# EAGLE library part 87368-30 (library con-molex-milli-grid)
RECEPTACAL
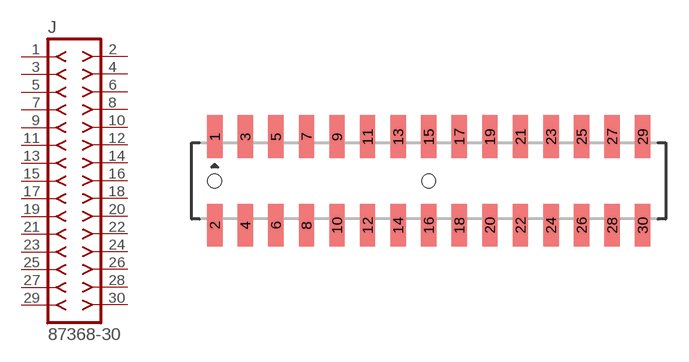
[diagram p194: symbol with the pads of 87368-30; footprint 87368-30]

Designator prefix J

## 87368-30  [87368-30]
1  1  pas
2  2  pas
3  3  pas
4  4  pas
5  5  pas
6  6  pas
7  7  pas
8  8  pas
9  9  pas
10  10  pas
11  11  pas
12  12  pas
13  13  pas
14  14  pas
15  15  pas
16  16  pas
17  17  pas
18  18  pas
19  19  pas
20  20  pas
21  21  pas
22  22  pas
23  23  pas
24  24  pas
25  25  pas
26  26  pas
27  27  pas
28  28  pas
29  29  pas
30  30  pas

## Footprint 87368-30 (pad centres in mm)
RECEPTACAL SMD Dual Row, Side Entry
smd 1 x 2.8: 1 -14,2.9; 2 -14,-2.9; 3 -12,2.9; 4 -12,-2.9; 5 -10,2.9; 6 -10,-2.9; 7 -8,2.9; 8 -8,-2.9; 9 -6,2.9; 10 -6,-2.9; 11 -4,2.9; 12 -4,-2.9; 13 -2,2.9; 14 -2,-2.9; 15 0,2.9; 16 0,-2.9; 17 2,2.9; 18 2,-2.9; 19 4,2.9; 20 4,-2.9; 21 6,2.9; 22 6,-2.9; 23 8,2.9; 24 8,-2.9; 25 10,2.9; 26 10,-2.9; 27 12,2.9; 28 12,-2.9; 29 14,2.9; 30 14,-2.9
hole 0.914 at -14,0
hole 0.914 at 0,0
